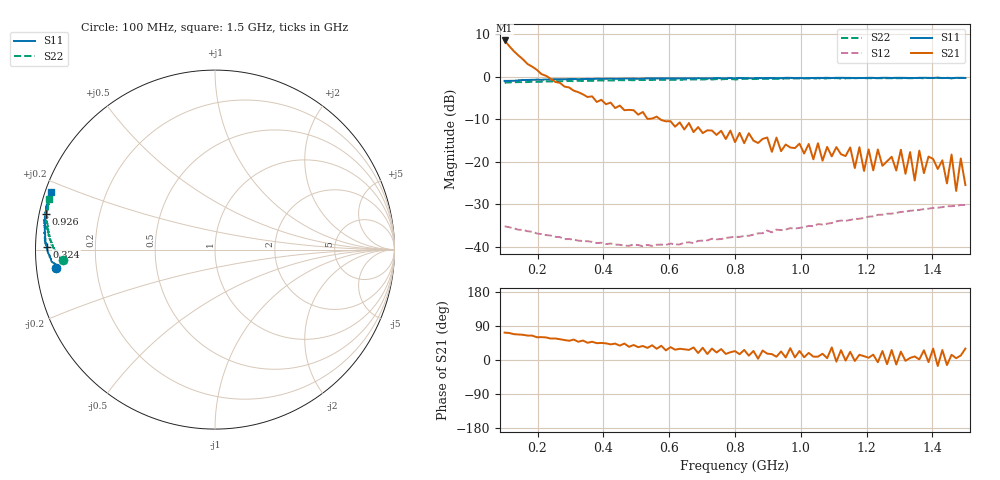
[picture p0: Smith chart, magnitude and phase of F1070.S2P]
!  POLYFET RF DEVICES
!  S PARAMETERS FOR
!  F1070 (Each Side)
!  VDS=28, IDQ=800mA
! Date: Nov 11, 1991
! Bias (V mA) : V1=3.5470000  I1=0.0070885  V2=27.990760  I2=768.13320
# MHZ S MA R 50
!  FREQ  S11 MAG  S11 ANG  S21 MAG  S21 ANG  S12 MAG  S12 ANG  S22 MAG  S22 ANG
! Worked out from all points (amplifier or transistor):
!   101 points, 100 MHz to 1.5 GHz, reference 50 ohm
!   highest |S21| = 8.5 dB at 100 MHz (marker M1)
!   |S21| within 3 dB of that: start of sweep to 134.8 MHz
!   unconditionally stable (mu >= 1): 353.3 MHz to 953.8 MHz; 954.3 MHz to 1.048 GHz; 1.115 GHz to 1.176 GHz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
!   at 324 MHz: K = 1.05, MAG = 16.0 dB, |S12| = -38.5 dB
!   at 800 MHz: K = 2.48, MAG = 4.4 dB, |S12| = -37.6 dB
!   at 1.5 GHz: K = 1.89, MAG = -3.1 dB, |S12| = -30.1 dB
!   S11 on the Smith chart (normalised r, x): 100 MHz: 0.06, -0.06; 324 MHz: 0.03, +0.01; 926 MHz: 0.02, +0.10; 1.5 GHz: 0.02, +0.17
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100  0.8929 -173.3  2.665 72.3  0.0175 -9.8  0.8504 -176.2
170  0.915 -176.7  1.407 64.4  0.0153 -9.8  0.8647 -177.5
324  0.9343 179.1  0.6583 48.2  0.01187 -2.4  0.8945 -180.0
338  0.9385 178.7  0.6205 51.3  0.01177 -2.3  0.8904 179.9
576  0.9524 174.1  0.3097 37.5  0.01067 26.9  0.9179 176.5
800  0.9576 170.3  0.1705 23.4  0.01319 47.8  0.9295 172.9
926  0.9611 168.1  0.1925 8.7  0.016 54.3  0.9485 171.3
1038  0.965 166.5  0.1071 8.8  0.01754 60.1  0.9513 169.8
1276  0.966 163.2  0.1147 26.3  0.02465 64.5  0.9581 166.6
1290  0.9713 163.3  0.0792 -12.0  0.02513 63.9  0.9614 165.7
1304  0.97 163.1  0.1387 22.0  0.02581 63.5  0.958 165.9
1318  0.9681 162.9  0.07244 -2.2  0.02599 63.7  0.963 165.6
1332  0.9642 162.6  0.1302 5.4  0.02665 64.7  0.9604 165.6
1346  0.9653 162.5  0.06041 9.4  0.02689 63.5  0.9612 165.0
1360  0.9698 162.6  0.1355 1.4  0.02726 63.4  0.9664 165.2
1374  0.9733 162.3  0.07365 25.6  0.02783 62.1  0.9587 164.7
1430  0.9639 161.8  0.1042 26.3  0.02936 62.9  0.9634 164.4
1444  0.9673 161.2  0.05576 -13.4  0.03011 61.3  0.9722 163.8
1458  0.9574 161.1  0.122 13.7  0.03013 62.2  0.9615 164.0
1472  0.9703 160.5  0.04543 4.8  0.03047 61.5  0.9662 163.4
1486  0.968 160.8  0.1096 11.9  0.03106 60.6  0.9697 163.5
1500  0.9667 160.8  0.05336 30.1  0.03111 61.0  0.9658 162.9
